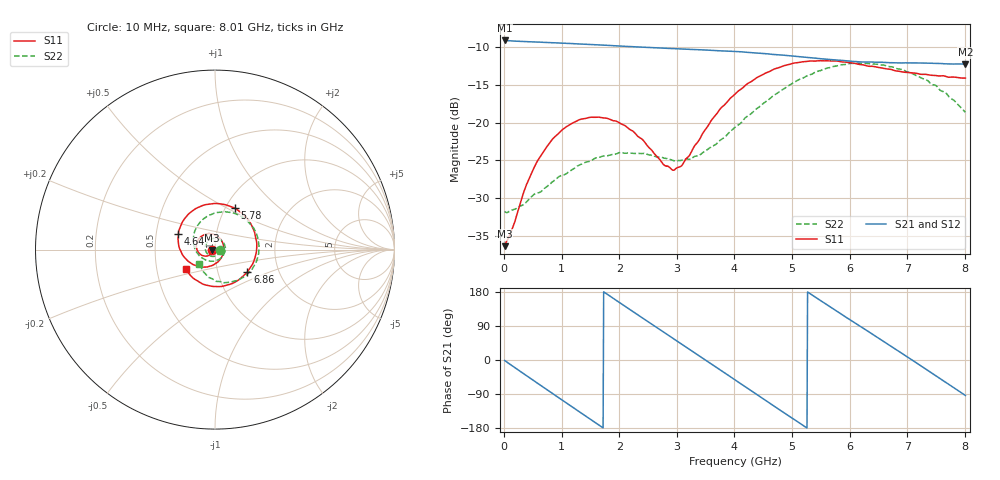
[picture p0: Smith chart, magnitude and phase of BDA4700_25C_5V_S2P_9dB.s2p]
!Agilent Technologies,E5071B,MY42404982,A.09.10
!Date: Mon Oct 20 13:30:31 2025
!Data & Calibration Information:
!Freq	S11:SOLT2(ON)	S21:SOLT2(ON)	S12:SOLT2(ON)	S22:SOLT2(ON)
# Hz S RI R 50
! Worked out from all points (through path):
!   801 points, 10 MHz to 8.01 GHz, reference 50 ohm
!   highest |S21| = -9.12 dB at 10 MHz (marker M1); lowest = -12.3 dB at 8.01 GHz (marker M2)
!   group delay of S21, straight-line fit = 281 ps
!   lowest |S11| = -36.4 dB at 10 MHz (marker M3), VSWR 1.03, Z = 48.5 - j0.142 ohm
!   |S11| at or under -10 dB: start of sweep to end of sweep
!   |S22| runs from -32.0 to -12.1 dB; largest |S21 - S12| = 0.0027
!   S11 on the Smith chart (normalised r, x): 10 MHz: 0.97, -0.00; 4.64 GHz: 0.65, +0.12; 5.78 GHz: 1.11, +0.55; 6.86 GHz: 1.39, -0.36; 8.01 GHz: 0.70, -0.16
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1e7  -0.0151 -0.00146  0.3498 -0.00745  0.3497 -0.00788  0.0257 -0.00141
4.2e8  -0.0291 -0.0291  0.2452 -0.2404  0.2452 -0.2408  0.0178 -0.025
7.1e8  -0.0553 -0.0364  0.0898 -0.3277  0.0896 -0.3279  -0.00149 -0.0368
1.02e9  -0.0875 -0.0215  -0.0973 -0.3212  -0.0974 -0.3214  -0.0302 -0.0331
1.35e9  -0.1043 0.0168  -0.2573 -0.2084  -0.2576 -0.2085  -0.0529 -0.00397
1.93e9  -0.0589 0.0838  -0.3017 0.114  -0.3017 0.1142  -0.0233 0.057
2.32e9  0.000601 0.0811  -0.1557 0.2759  -0.1558 0.2759  0.0264 0.0567
2.68e9  0.0418 0.0404  0.0387 0.3099  0.0387 0.3099  0.056 0.0186
2.96e9  0.0477 -0.00896  0.1794 0.251  0.1794 0.2508  0.0526 -0.0186
3.37e9  0.00781 -0.0745  0.2962 0.0675  0.2966 0.0672  0.0117 -0.059
3.68e9  -0.0566 -0.0974  0.2839 -0.0961  0.284 -0.0969  -0.0362 -0.0618
4.01e9  -0.1343 -0.0756  0.1803 -0.2344  0.1805 -0.2342  -0.0855 -0.036
4.33e9  -0.1908 -0.00797  0.0251 -0.2887  0.0248 -0.2892  -0.1167 0.0191
4.64e9  -0.2038 0.0855  -0.1279 -0.253  -0.1276 -0.2534  -0.1163 0.0892
5.01e9  -0.1505 0.1951  -0.2482 -0.1197  -0.2488 -0.1199  -0.0653 0.1702
5.35e9  -0.0456 0.2515  -0.2652 0.0401  -0.2655 0.0394  0.0272 0.2081
5.78e9  0.1116 0.2302  -0.1618 0.2029  -0.1615 0.203  0.1596 0.1759
6.21e9  0.2162 0.1079  0.0156 0.2515  0.0178 0.2517  0.24 0.057
6.68e9  0.2162 -0.0657  0.1912 0.1602  0.1917 0.1601  0.2161 -0.0929
6.86e9  0.1807 -0.1231  0.2299 0.0938  0.2303 0.0928  0.1793 -0.1383
7.36e9  0.0245 -0.2061  0.2189 -0.1154  0.219 -0.1157  0.044 -0.184
8.01e9  -0.1637 -0.1096  -0.0151 -0.2433  -0.0147 -0.2436  -0.0864 -0.0789
